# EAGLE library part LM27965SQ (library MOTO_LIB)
LED driver LM27965
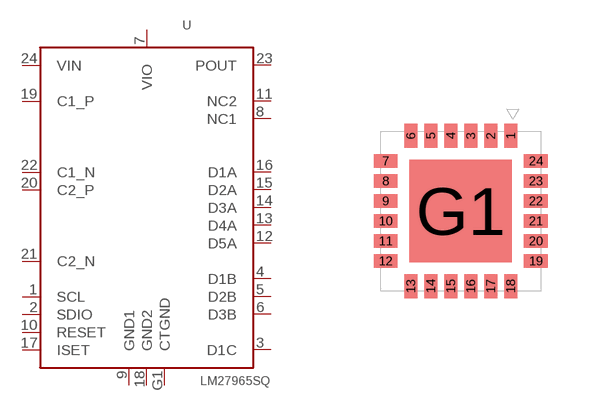
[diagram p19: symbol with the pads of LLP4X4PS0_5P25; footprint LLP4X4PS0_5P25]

Designator prefix U

## LM27965SQ (MPN: LM27965SQ; SUPPLIER: TI)  [LLP4X4PS0_5P25]
1  SCL
2  SDIO
3  D1C
4  D1B
5  D2B
6  D3B
7  VIO
8  NC1
9  GND1
10  RESET
11  NC2
12  D5A
13  D4A
14  D3A
15  D2A
16  D1A
17  ISET
18  GND2
19  C1_P
20  C2_P
21  C2_N
22  C1_N
23  POUT
24  VIN
G1  CTGND

## Footprint LLP4X4PS0_5P25 (pad centres in mm)
smd 0.33 x 0.6: 1 1.25,1.88; 2 0.75,1.88; 3 0.25,1.88; 4 -0.25,1.88; 5 -0.75,1.88; 6 -1.25,1.88; 13 -1.25,-1.88; 14 -0.75,-1.88; 15 -0.25,-1.88; 16 0.25,-1.88; 17 0.75,-1.88; 18 1.25,-1.88
smd 0.6 x 0.33: 7 -1.88,1.25; 8 -1.88,0.75; 9 -1.88,0.25; 10 -1.88,-0.25; 11 -1.88,-0.75; 12 -1.88,-1.25; 19 1.88,-1.25; 20 1.88,-0.75; 21 1.88,-0.25; 22 1.88,0.25; 23 1.88,0.75; 24 1.88,1.25
smd 2.56 x 2.56: G1 0,0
